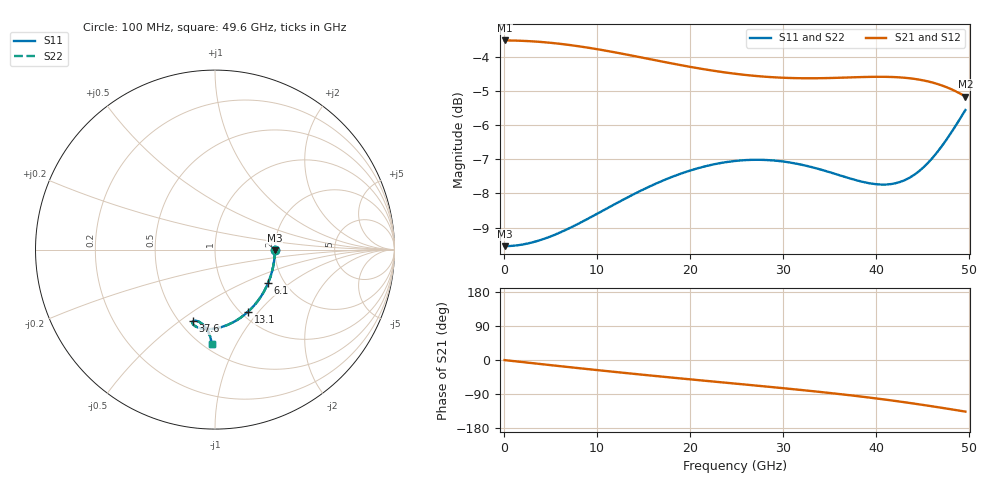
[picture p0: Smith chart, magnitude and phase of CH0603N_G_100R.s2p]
# GHz S RI R 100
! S-Parameters data
! Freq  reS11  imS11  reS21  imS21  reS12  imS12  reS22  imS22
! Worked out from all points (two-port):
!   100 points, 100 MHz to 49.6 GHz, reference 100 ohm
!   highest |S21| = -3.52 dB at 100 MHz (marker M1); lowest = -5.2 dB at 49.6 GHz (marker M2)
!   |S21| within 3 dB of the highest: start of sweep to end of sweep
!   lowest |S11| = -9.5 dB at 100 MHz (marker M3), VSWR 2.00, Z = 200 - j1.41 ohm
!   |S11| at or under -10 dB: nowhere
!   |S22| runs from -9.5 to -5.6 dB; largest |S21 - S12| = 0
!   S11 on the Smith chart (normalised r, x): 100 MHz: 2.00, -0.01; 6.1 GHz: 1.66, -0.70; 13.1 GHz: 1.08, -0.88; 37.6 GHz: 0.58, -0.56; 49.6 GHz: 0.55, -0.80
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0.1  0.3333 -0.00314  0.6667 -0.00314  0.6667 -0.00314  0.3333 -0.00314
3.1  0.3236 -0.0964  0.6576 -0.0966  0.6576 -0.0966  0.3236 -0.0964
6.1  0.2968 -0.1841  0.6324 -0.1856  0.6324 -0.1856  0.2968 -0.1841
8.6  0.2633 -0.2498  0.6007 -0.2538  0.6007 -0.2538  0.2633 -0.2498
11.1  0.222 -0.3066  0.5611 -0.3152  0.5611 -0.3152  0.222 -0.3066
13.1  0.1851 -0.345  0.5252 -0.3589  0.5252 -0.3589  0.1851 -0.345
16.6  0.1164 -0.3962  0.456 -0.4238  0.456 -0.4238  0.1164 -0.3962
18.6  0.0768 -0.4165  0.4141 -0.4547  0.4141 -0.4547  0.0768 -0.4165
20.6  0.0384 -0.4307  0.3712 -0.4816  0.3712 -0.4816  0.0384 -0.4307
22.6  0.00213 -0.4392  0.3276 -0.5049  0.3276 -0.5049  0.00213 -0.4392
25.1  -0.0388 -0.4428  0.272 -0.5296  0.272 -0.5296  -0.0388 -0.4428
29.1  -0.0907 -0.4354  0.1801 -0.5606  0.1801 -0.5606  -0.0907 -0.4354
31.1  -0.1087 -0.4274  0.1319 -0.5723  0.1319 -0.5723  -0.1087 -0.4274
33.1  -0.1206 -0.418  0.0815 -0.5812  0.0815 -0.5812  -0.1206 -0.418
35.6  -0.1259 -0.4062  0.0145 -0.5875  0.0145 -0.5875  -0.1259 -0.4062
37.6  -0.1221 -0.399  -0.0429 -0.5873  -0.0429 -0.5873  -0.1221 -0.399
39.6  -0.1112 -0.3961  -0.1038 -0.5805  -0.1038 -0.5805  -0.1112 -0.3961
41.6  -0.0939 -0.4  -0.1675 -0.5652  -0.1675 -0.5652  -0.0939 -0.4
43.6  -0.0722 -0.4135  -0.2325 -0.5389  -0.2325 -0.5389  -0.0722 -0.4135
45.6  -0.0492 -0.4389  -0.2955 -0.4998  -0.2955 -0.4998  -0.0492 -0.4389
47.6  -0.0295 -0.4771  -0.3525 -0.4471  -0.3525 -0.4471  -0.0295 -0.4771
49.6  -0.0183 -0.5271  -0.3983 -0.382  -0.3983 -0.382  -0.0183 -0.5271
